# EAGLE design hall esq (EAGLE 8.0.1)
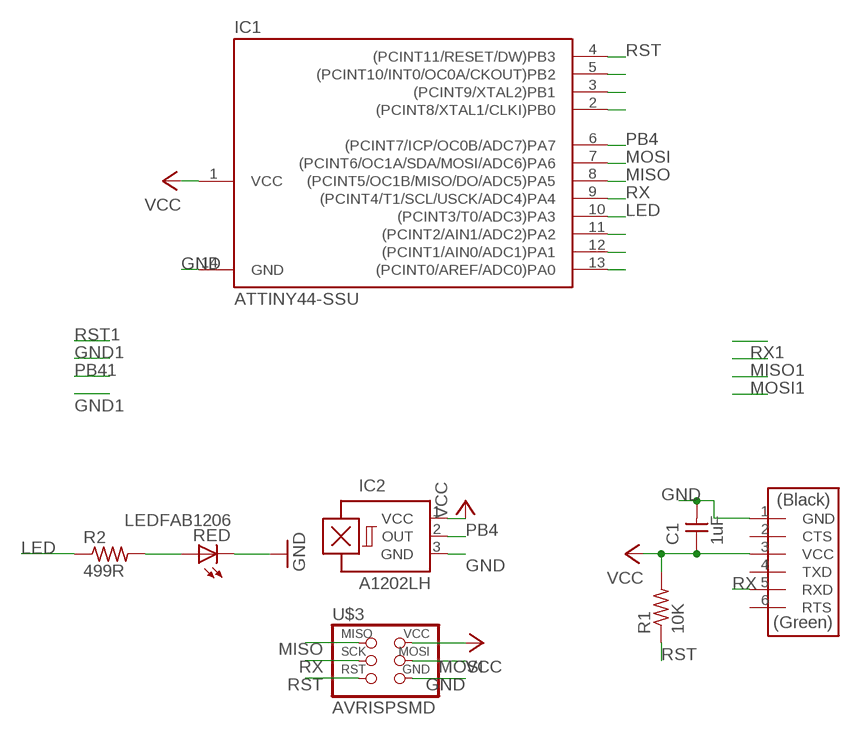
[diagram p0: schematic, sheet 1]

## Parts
C1  1uF  CAP-UNPOLARIZEDFAB  [C1206FAB]
IC1  ATTINY44-SSU  [SOIC14]
IC2  A1202LH  [SOT23-W]
R1  10K  RES-US1206FAB  [R1206FAB]
R2  499R  RES-US1206FAB  [R1206FAB]
RED  LEDFAB1206  [LED1206FAB]
U$2  FTDI-SMD-HEADER  [1X06SMD]
U$3  AVRISPSMD  [2X03SMD]

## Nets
GND: C1.2 IC1.14(GND) IC2.3(GND) RED.2(C) U$2.1(GND) U$3.6(GND)
LED: IC1.10((PCINT3/T0/ADC3)PA3) R2.1
MISO: IC1.8((PCINT5/OC1B/MISO/DO/ADC5)PA5) U$3.1(MISO)
MOSI: IC1.7((PCINT6/OC1A/SDA/MOSI/ADC6)PA6) U$3.4(MOSI)
N$1: R2.2 RED.1(A)
N$4: IC1.5((PCINT10/INT0/OC0A/CKOUT)PB2)
N$5: IC1.3((PCINT9/XTAL2)PB1)
N$6: IC1.2((PCINT8/XTAL1/CLKI)PB0)
N$12: IC1.11((PCINT2/AIN1/ADC2)PA2)
N$13: IC1.12((PCINT1/AIN0/ADC1)PA1)
N$14: IC1.13((PCINT0/AREF/ADC0)PA0)
PB4: IC1.6((PCINT7/ICP/OC0B/ADC7)PA7) IC2.2(OUT)
RST: IC1.4((PCINT11/RESET/DW)PB3) R1.1 U$3.5(RST)
RX: IC1.9((PCINT4/T1/SCL/USCK/ADC4)PA4) U$2.5(RXD) U$3.3(SCK)
VCC: C1.1 IC1.1(VCC) IC2.1(VCC) R1.2 U$2.3(VCC) U$3.2(VCC)
Unconnected: U$2.2(CTS) U$2.4(TXD) U$2.6(RTS)

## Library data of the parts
C1 = fab:CAP-UNPOLARIZED
IC1 = fab:ATTINY44
IC2 = allegro:A12*?: Hall-effect bipolar switch Source: http://www.allegromicro.com/en/Products/Part_Numbers/1202/1202.pdf; OC_FARNELL: unknown; OC_NEWARK: unknown
R1 R2 = fab:RES-US: Resistor (US Symbol)
RED = fab:LED: LED
U$2 = fab:FTDI-SMD-HEADER
U$3 = fab:AVRISP

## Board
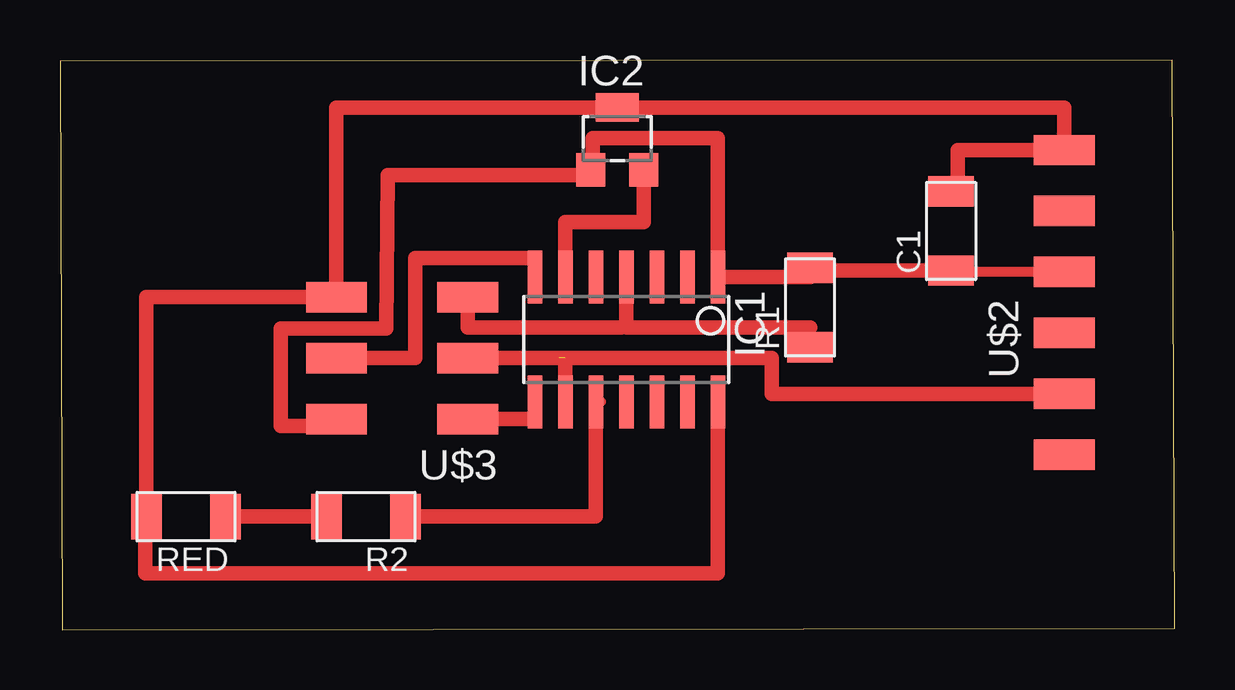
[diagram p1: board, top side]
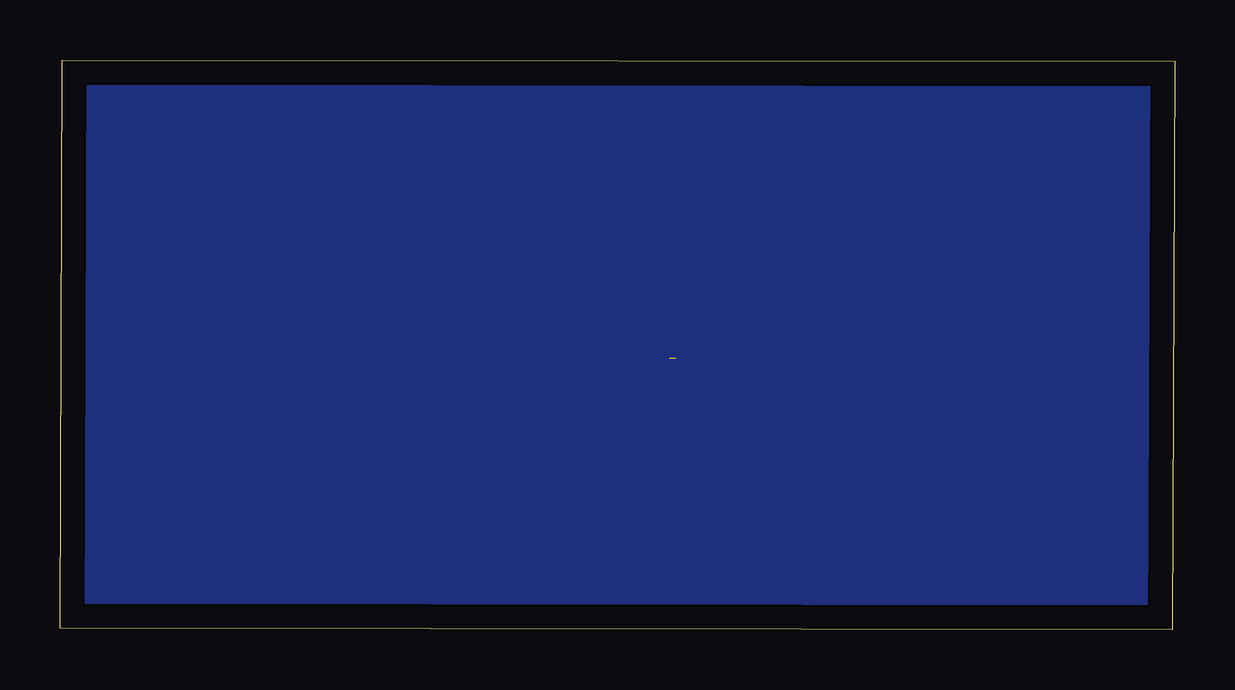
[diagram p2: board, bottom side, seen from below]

Size 46.45 x 23.75 mm. Coordinates in mm from the lower left corner, seen from the top.
Outline: 0.1,0 46.45,0.05 46.35,23.75 0,23.7 0.1,0
Copper layers (1*16): Top 0.035mm / dielectric 1.5mm / Bottom 0.035mm
Design rules "default": minimum track width 10mil, minimum drill 24mil, track to track 8mil, track to pad 8mil, pad to pad 8mil, via to via 8mil, smd to smd 8mil, copper to edge 40mil, drill to drill 8mil, minimum pad ring 10mil, minimum via ring 8mil, stop-mask expansion 4mil, vias tented up to drill 0mil, thermal gap 10mil

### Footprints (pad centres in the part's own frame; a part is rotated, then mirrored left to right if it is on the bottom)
C1206FAB = smd 1.27 x 1.905: 1 -1.651,0; 2 1.651,0
SOIC14 = smd 0.61 x 2.21: 1 -3.81,-2.603; 2 -2.54,-2.603; 3 -1.27,-2.603; 4 0,-2.603; 5 1.27,-2.603; 6 2.54,-2.603; 7 3.81,-2.603; 8 3.81,2.603; 9 2.54,2.603; 10 1.27,2.603; 11 0,2.603; 12 -1.27,2.603; 13 -2.54,2.603; 14 -3.81,2.603
SOT23-W = smd 1.2 x 1.4: 1 -1.1,-1.3; 2 1.1,-1.3 | smd 1.8 x 1.2: 3 0,1.3
R1206FAB = smd 1.27 x 1.905: 1 -1.651,0; 2 1.651,0
LED1206FAB = smd 1.27 x 1.905: 1 -1.651,0; 2 1.651,0
1X06SMD = smd 2.54 x 1.27: 1 0,6.35; 2 0,3.81; 3 0,1.27; 4 0,-1.27; 5 0,-3.81; 6 0,-6.35
2X03SMD = smd 2.54 x 1.27: 1 -2.54,2.54; 2 2.92,2.54; 3 -2.54,0; 4 2.92,0; 5 -2.54,-2.54; 6 2.92,-2.54

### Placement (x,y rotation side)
C1  37.13,16.62 90 top
IC1  23.6,12.1 180 top
IC2  23.22,20.47 0 top
R1  31.25,13.43 90 top
R2  12.75,4.71 180 top
RED  5.25,4.71 180 top
U$2  41.85,13.64 0 top
U$3  14.44,11.32 180 top

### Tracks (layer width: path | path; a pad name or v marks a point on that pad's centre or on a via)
GND
  Top 0.406: C1.2 37.4,18.27 | 3.55,4.71 RED.2
  Top 0.61: 37.4,18.27 37.4,19.99 U$2.1 41.85,21.77 IC2.3 11.52,21.77 U$3.6 3.6,13.86 RED.2 | IC1.14 27.41,2.35 3.55,2.35 3.55,4.71
LED
  Top 0.406: 22.55,9.5 IC1.10 22.45,9.5 | 14.4,4.66 R2.1 14.4,4.5
  Top 0.61: R2.1 22.33,4.71 IC1.10
MISO
  Top 0.406: 19.79,8.78 IC1.8
  Top 0.61: 19.79,8.78 U$3.1
MOSI
  Top 0.406: IC1.7 19.79,15.5
  Top 0.61: 19.79,15.5 14.8,15.5 14.8,11.32 U$3.4
N$1
  Top 0.61: R2.2 RED.1
N$2
  pour Bottom: 0.1,22.8 45.7,22.8 45.7,0 0.1,0
N$7
  pour Bottom: 1.1,1 1.1,22.5 44.6,22.5 44.6,1
PB4
  Top 0.61: IC1.6 21.06,17 24.32,17 IC2.2
RST
  Top 0.406: 23.4,12.6 23.6,12.6 | 31.25,12.6 R1.1
  Top 0.61: IC1.4 23.6,12.6 31.25,12.6 | U$3.5 16.98,12.6 23.4,12.6
RX  (1 unrouted)
  Top 0.406: IC1.9
  Top 0.61: U$3.3 21.06,11.32 IC1.9 | 20.8,11.32 29.65,11.32 29.65,9.83 U$2.5
VCC
  Top 0.406: U$2.3 37.13,14.91 C1.1 | 27.41,14.23 IC1.1 | 22.17,18.95 IC2.1 22.2,19.17 | 11.52,8.5 U$3.2 | 31.25,14.7 R1.2 31.25,14.97
  Top 0.61: C1.1 31.25,14.97 | 11.52,8.5 9.2,8.5 9.2,12.55 13.6,12.55 13.65,18.95 22.17,18.95 | 31.25,14.7 IC1.1 27.41,20.5 22.2,20.5 22.2,19.17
